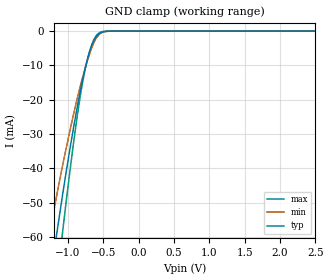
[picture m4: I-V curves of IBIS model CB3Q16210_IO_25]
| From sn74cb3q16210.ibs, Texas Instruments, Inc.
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[Model]   CB3Q16210_IO_25
Model_type  Terminator
| variable   typ   min   max
C_comp   3.36pF   2.77pF   3.97pF
| C_tri-state   3.36pF   2.77pF   3.97pF
[Temperature Range]   40   100   -40
| Ambient temperature   25   85   -40
[Voltage range]   2.5   2.3   2.7
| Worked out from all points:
|   GND clamp passes 1 mA (typ) near -0.57 V on its own axis
[GND Clamp]
| CB3Q16210_IO_25
|   Voltage   I(typ)   I(min)   I(max)
-5.5V     -867.9mA   -713.7mA   -1.031A
-1.25V    -72.16mA   -57.85mA   -90.64mA
-1.155V   -58.52mA   -47.44mA   -72.8mA
-1.075V   -47.57mA   -39.09mA   -58.36mA
-910mV    -26.85mA   -23.26mA   -30.89mA
-790mV    -13.95mA   -13.25mA   -14.58mA
-730mV    -8.588mA   -8.918mA   -8.785mA
-670mV    -4.456mA   -5.245mA   -4.445mA
-620mV    -2.23mA    -2.86mA    -2.012mA
-560mV    -793.9uA   -1.037mA   -543.8uA
-340mV    -2.999uA   -5.303uA   -306.5nA
2.5V      108.4pA    476.7pA    26.76pA
